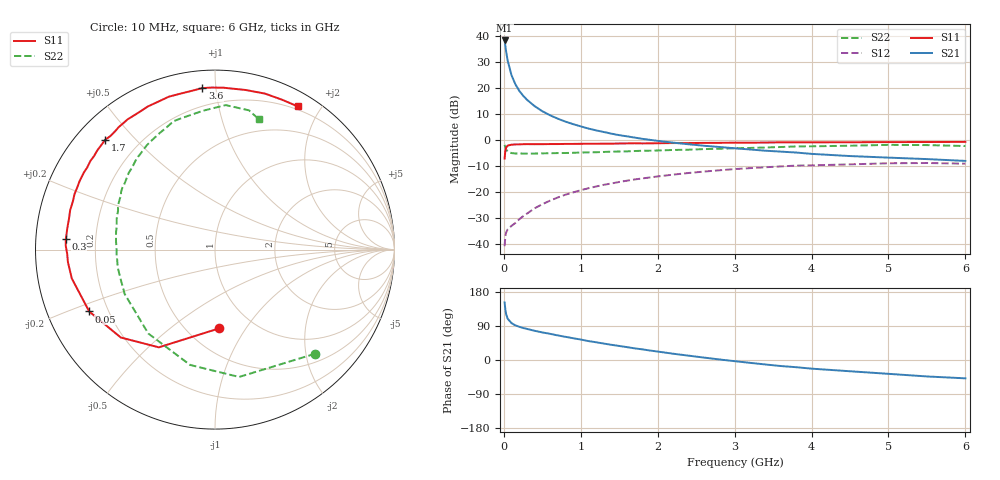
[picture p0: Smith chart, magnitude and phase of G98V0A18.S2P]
! SIEMENS Small Signal Semiconductors
! BFG235
! Si NPN RF Bipolar Junction Transistor in SOT223
! VCE = 8 V  IC = 180 mA
! Common Emitter S-Parameters:  July  1994
# GHz  S  MA  R  50
!  f  S11  S21  S12  S22
! GHz  MAG  ANG  MAG  ANG  MAG  ANG  MAG  ANG
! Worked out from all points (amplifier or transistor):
!   40 points, 10 MHz to 6 GHz, reference 50 ohm
!   highest |S21| = 38.4 dB at 10 MHz (marker M1)
!   |S21| within 3 dB of that: start of sweep to 24.05 MHz
!   unconditionally stable (mu >= 1): 454.5 MHz to 1.501 GHz
!   at 200 MHz: K = 0.81, MSG = 24.8 dB, |S12| = -30.5 dB
!   at 1.5 GHz: K = 1.00, MAG = 9.0 dB, |S12| = -16.2 dB
!   at 6 GHz: K = 0.89, MSG = 0.5 dB, |S12| = -9.1 dB
!   S11 on the Smith chart (normalised r, x): 10 MHz: 0.70, -0.77; 50 MHz: 0.13, -0.23; 300 MHz: 0.09, +0.03; 1.7 GHz: 0.08, +0.41; 3.6 GHz: 0.09, +0.92; 6 GHz: 0.16, +1.72
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0.01  0.4394 -86.9  83.02 151.9  0.009 60.9  0.805 -46.1
0.02  0.6281 -119.9  65.03 132.9  0.0141 47.7  0.7222 -79.3
0.03  0.718 -137.0  50.66 121.2  0.0165 41.2  0.6574 -102.2
0.05  0.781 -153.8  33.62 108.9  0.019 34.2  0.5972 -128.5
0.1  0.8139 -168.6  17.72 97.2  0.0222 37.4  0.5607 -153.8
0.15  0.8224 -175.1  11.88 91.4  0.0252 44.1  0.5505 -164.3
0.2  0.824 -178.4  8.896 87.7  0.0297 48.9  0.551 -169.9
0.25  0.8316 178.6  7.166 84.5  0.0339 52.3  0.548 -173.7
0.3  0.8332 176.0  5.983 82.0  0.0381 55.5  0.5487 -176.9
0.4  0.8314 171.6  4.501 77.1  0.0483 58.7  0.5488 178.9
0.5  0.8316 167.9  3.594 72.8  0.0579 60.3  0.553 175.5
0.6  0.8364 164.8  3.002 69.1  0.0678 60.4  0.5567 172.3
0.8  0.8416 158.4  2.266 61.2  0.0883 59.6  0.562 167.1
1.1  0.8476 149.5  1.661 49.9  0.1178 55.8  0.5785 160.2
1.4  0.8517 142.4  1.326 40.1  0.1457 51.1  0.5962 154.1
1.7  0.8655 135.0  1.114 30.7  0.1739 45.8  0.6139 148.5
2.2  0.8738 123.8  0.891 16.6  0.2153 36.6  0.6432 138.4
3.2  0.8899 102.6  0.657 -7.5  0.2871 17.3  0.7041 119.8
3.6  0.9026 94.5  0.598 -15.9  0.3101 8.9  0.7334 111.4
4.5  0.9055 79.1  0.491 -29.7  0.3396 -7.4  0.7766 94.9
5.5  0.9149 65.8  0.429 -43.4  0.3605 -25.7  0.7987 76.3
6  0.9213 60.0  0.396 -48.4  0.3503 -32.6  0.766 71.4
